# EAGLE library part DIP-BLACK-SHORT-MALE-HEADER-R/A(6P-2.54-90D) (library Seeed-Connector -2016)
320020019
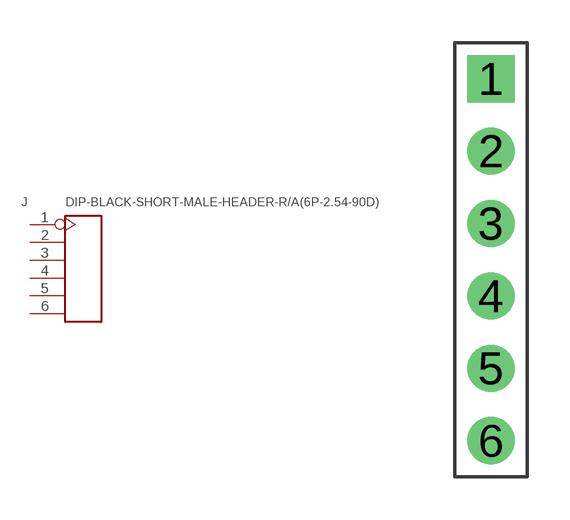
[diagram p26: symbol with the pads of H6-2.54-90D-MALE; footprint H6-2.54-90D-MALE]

Designator prefix J

## DIP-BLACK-SHORT-MALE-HEADER-R/A(6P-2.54-90D) (VALUE: 6p-2.54-90d)  [H6-2.54-90D-MALE]
1  1
2  2
3  3
4  4
5  5
6  6

## Footprint H6-2.54-90D-MALE (pad centres in mm)
drill 0.889 pad 1.651 square: 1 0,6.35
drill 0.889 pad 1.651: 2 0,3.81; 3 0,1.27; 4 0,-1.27; 5 0,-3.81; 6 0,-6.35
